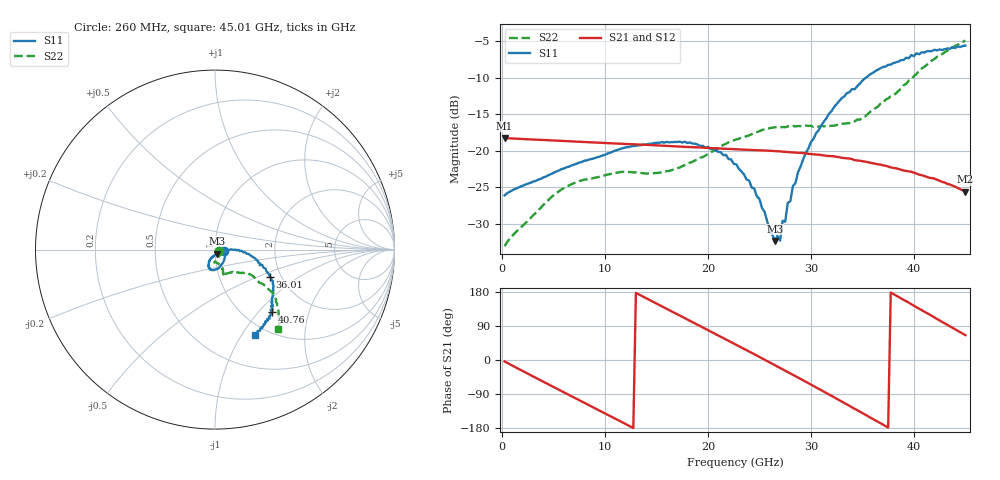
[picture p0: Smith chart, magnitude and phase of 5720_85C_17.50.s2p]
! Device:  ADRF5720
! Description: 0.5dB LSB GaAs MMIC 6-bit Digital Attenuator
! Frequency:  0.000009 -  40 GHz
! Ports:
!	RF1	= Port 1
!	RF2	= Port 2
! Vdd:  3.3 Volt
! Vss:  -3.3 Volt
! Control:  0/3.3 Volt
! State:  17.50 dB attenuation
! Data:  The device was measured using G-S-G Probes on a matrix board.
!  Data was collected using an calibrated 4 port network analyzer.
!  The reference plane for this measurement is at the launchers.
! Note:  Analog Devices supplies this data as a sample of measured data
!  for this product.  Your particular data for this product may vary.
!  Data was taken at 85 degrees C.
!  Analog Devices reserves the right to change this data at anytime.
# GHZ S DB R 45.0
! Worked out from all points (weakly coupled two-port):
!   180 points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, 260 MHz to 45.01 GHz, reference 45 ohm
!   highest |S21| = -18.26 dB at 260 MHz (marker M1); lowest = -25.6 dB at 45.01 GHz (marker M2)
!   lowest |S11| = -32.3 dB at 26.51 GHz (marker M3), VSWR 1.05, Z = 45.9 - j2.01 ohm
!   |S11| at or under -10 dB: start of sweep to 35.36 GHz
!   |S22| runs from -33.0 to -4.9 dB; largest |S21 - S12| = 0.00066
!   S11 on the Smith chart (normalised r, x): 260 MHz: 1.10, -0.02; 36.01 GHz: 1.75, -0.60; 40.76 GHz: 1.33, -1.19; 45.01 GHz: 0.87, -1.14
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0.26  -26.10 -10.4  -18.26 -3.9  -18.26 -3.9  -33.04 -22.0
5.01  -23.01 -39.8  -18.59 -71.2  -18.58 -71.2  -26.09 -67.8
7.76  -21.53 -57.1  -18.78 -109.6  -18.77 -109.6  -24.05 -82.9
11.76  -19.65 -78.2  -19.05 -165.4  -19.04 -165.3  -22.89 -92.8
15.26  -18.90 -92.8  -19.27 145.4  -19.26 145.6  -23.00 -86.9
20.01  -19.47 -108.6  -19.60 78.8  -19.58 79.0  -20.45 -70.4
22.76  -21.86 -114.3  -19.80 40.0  -19.78 40.2  -18.47 -68.9
24.51  -25.17 -113.5  -19.91 15.2  -19.90 15.5  -17.59 -70.5
26.51  -32.33 -64.9  -20.05 -13.6  -20.03 -13.4  -16.77 -70.7
26.76  -31.63 -51.1  -20.06 -17.3  -20.05 -17.0  -16.79 -71.0
27.01  -32.29 -36.6  -20.08 -20.9  -20.07 -20.7  -16.79 -70.5
27.26  -29.58 -25.0  -20.12 -24.7  -20.11 -24.4  -16.75 -71.2
27.51  -29.69 -16.6  -20.15 -28.2  -20.14 -27.9  -16.78 -70.6
27.76  -27.12 -11.8  -20.17 -31.9  -20.16 -31.6  -16.66 -71.4
28.01  -26.90 -8.6  -20.21 -35.6  -20.20 -35.3  -16.70 -71.1
28.26  -24.82 -4.9  -20.23 -39.1  -20.22 -38.8  -16.61 -71.6
30.26  -18.37 -2.2  -20.48 -68.5  -20.46 -68.3  -16.73 -69.4
33.01  -12.80 -12.4  -20.96 -109.9  -20.94 -109.6  -16.31 -58.6
36.01  -9.37 -26.3  -21.70 -155.4  -21.68 -155.1  -14.47 -43.1
37.76  -8.23 -33.5  -22.27 177.9  -22.25 178.2  -12.55 -35.6
40.76  -6.53 -47.5  -23.33 131.7  -23.30 132.1  -8.76 -36.5
45.01  -5.61 -65.0  -25.58 65.7  -25.55 66.0  -4.92 -51.6
